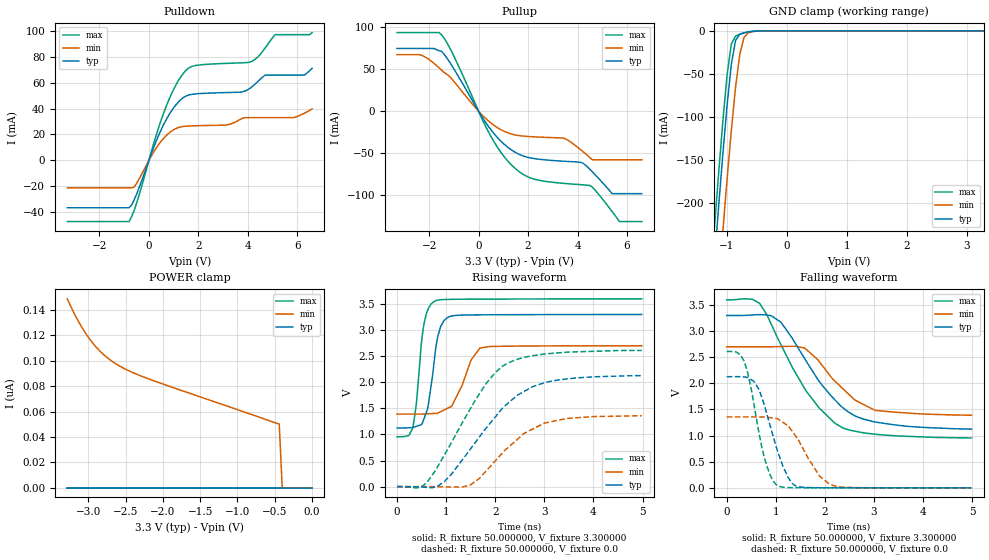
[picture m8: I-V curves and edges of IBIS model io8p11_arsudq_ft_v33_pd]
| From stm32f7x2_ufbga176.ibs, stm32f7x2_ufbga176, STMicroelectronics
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|   Model io8p11_arsudq_ft_v33_pd
[Model]  io8p11_arsudq_ft_v33_pd
Model_type I/O
Polarity   Non-Inverting
Enable   Active-Low
Vinl =   0.990000V
Vinh =   2.310000V
Vmeas =  1.650000V
Cref =   30.000000pF
Rref =   100.000000M
Vref =   0.0V
C_comp   2.292100pF   2.219400pF   2.369900pF
[Temperature Range]   25.000000   0.125000k   -40.000000
[Pullup Reference]   3.300000V   2.700000V   3.600000V
[Pulldown Reference]   0.0V   0.0V   0.0V
[POWER Clamp Reference]   3.300000V   2.700000V   3.600000V
[GND Clamp Reference]   0.0V   0.0V   0.0V
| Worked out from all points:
|   slope of the pulldown table from 0 to 0.495 V, typ, clamps not added: 20.9 ohm
|   slope of the pullup table from 0 to 0.495 V, typ, clamps not added: 22.6 ohm
|   GND clamp passes 1 mA (typ) near -0.62 V on its own axis
|   rising waveform, R_fixture 50.000000, V_fixture 3.300000: 20-80 % time 192ps typ, 344ps min, 163ps max; typ from 1.12 V to 3.3 V
|   rising waveform, R_fixture 50.000000, V_fixture 0.0: 20-80 % time 1.13ns typ, 939ps min, 1ns max; typ from 0 V to 2.13 V
|   falling waveform, R_fixture 50.000000, V_fixture 3.300000: 20-80 % time 999ps typ, 803ps min, 996ps max; typ from 3.3 V to 1.12 V
|   falling waveform, R_fixture 50.000000, V_fixture 0.0: 20-80 % time 415ps typ, 530ps min, 330ps max; typ from 2.13 V to 0 V
[Pulldown]
|Voltage   I(typ)   I(min)   I(max)
-3.3V     -36.46mA   -21.1mA    -47.09mA
-800mV    -36.46mA   -21.1mA    -47.09mA
-600mV    -30.5mA    -20.54mA   -38.69mA
700mV     31.4mA     19.11mA    41.71mA
1.2V      45.15mA    25.37mA    61.75mA
1.6V      50.35mA    26.5mA     71.06mA
3.1V      52.27mA    27.26mA    74.75mA
4.1V      55.69mA    32.97mA    75.8mA
4.7V      65.7mA     32.97mA    86.63mA
5.1V      65.7mA     32.97mA    96.89mA
6.3V      65.87mA    36.5mA     96.89mA
6.6V      70.93mA    39.71mA    98.5mA
[Pullup]
|Voltage   I(typ)   I(min)   I(max)
-3.3V     74.73mA    67.41mA    93.64mA
-2.3V     74.73mA    66.57mA    93.64mA
-1.5V     71.36mA    49.01mA    91.06mA
-1V       50.51mA    35.49mA    65.51mA
500mV     -22.07mA   -14mA      -30.03mA
1.6V      -50.64mA   -28.81mA   -70.96mA
3.5V      -59.53mA   -32.65mA   -85.92mA
4.2V      -61.43mA   -47.47mA   -87.46mA
4.5V      -69.06mA   -55.01mA   -88.38mA
5.4V      -98mA      -57.7mA    -119.3mA
5.7V      -98mA      -57.7mA    -131.2mA
6.6V      -98mA      -57.7mA    -131.2mA
[GND_clamp]
|Voltage   I(typ)   I(min)   I(max)
-3.3V     -2.314A    -2.394A    -2.287A
-1.2V     -265.5mA   -356.1mA   -227.2mA
-1.13V    -202.7mA   -292.9mA   -164.1mA
-1.06V    -142.2mA   -231.2mA   -104.1mA
-990mV    -85.98mA   -171.6mA   -50.73mA
-920mV    -38.81mA   -115.5mA   -15.29mA
-850mV    -11.09mA   -65.61mA   -6.016mA
-780mV    -3.793mA   -27.42mA   -3.89mA
-710mV    -2.098mA   -7.698mA   -2.396mA
-640mV    -1.159mA   -2.127mA   -1.234mA
-570mV    -535.1uA   -807.4uA   -490.2uA
3.28V     81.28uA    57.87uA    93.98uA
[POWER_clamp]
|Voltage   I(typ)   I(min)   I(max)
-3.28V    0A         148.5nA    0A
-3.2V     0A         138.6nA    0A
-3.12V    0A         129.7nA    0A
-3.04V    0A         122nA      0A
-2.96V    0A         115.3nA    0A
-2.8V     0A         105.1nA    0A
-2.6V     0A         96.44nA    0A
-2.4V     0A         90.52nA    0A
-2.16V    0A         84.97nA    0A
-440mV    0A         50.04nA    0A
-400mV    0A         0A         0A
0V        0A         0A         0A
[Ramp]
| variable   typ   min   max
dV/dt_r  1.26618/1.12392n   0.80934/0.93457n   1.56192/1.00073n
dV/dt_f  1.28340/0.99053n   0.77868/0.79554n   1.57246/0.99434n
R_load = 50.000000
[Rising Waveform]
R_fixture= 50.000000
V_fixture= 3.300000
V_fixture_min= 2.700000
V_fixture_max= 3.600000
|time   V(typ)   V(min)   V(max)
0s        1.123V     1.391V     953.8mV
320.3ps   1.132V     1.39V      1.122V
550.6ps   1.305V     1.393V     3.124V
630.6ps   1.526V     1.397V     3.393V
750.8ps   2.348V     1.402V     3.544V
830.8ps   2.88V      1.409V     3.574V
961ps     3.185V     1.469V     3.585V
1.121ns   3.27V      1.554V     3.589V
1.692ns   3.292V     2.656V     3.593V
4.985ns   3.299V     2.699V     3.598V
[Rising Waveform]
R_fixture= 50.000000
V_fixture= 0.0
V_fixture_min= 0.0
V_fixture_max= 0.0
|time   V(typ)   V(min)   V(max)
0s        211.7uV    83uV       632.1uV
550.6ps   -11.3mV    -125.6uV   33.63mV
961ps     92.14mV    -4.256mV   600.2mV
1.491ns   716.3mV    30.14mV    1.49V
1.812ns   1.118V     297mV      1.973V
2.232ns   1.576V     724.6mV    2.355V
2.593ns   1.826V     1.023V     2.477V
3.013ns   1.994V     1.22V      2.542V
3.473ns   2.066V     1.308V     2.577V
4.985ns   2.127V     1.358V     2.61V
[Falling Waveform]
R_fixture= 50.000000
V_fixture= 3.300000
V_fixture_min= 2.700000
V_fixture_max= 3.600000
|time   V(typ)   V(min)   V(max)
0s        3.299V     2.699V     3.598V
520.5ps   3.308V     2.699V     3.608V
670.7ps   3.314V     2.699V     3.53V
1.101ns   3.172V     2.704V     2.746V
1.592ns   2.467V     2.672V     1.893V
1.882ns   2.04V      2.418V     1.53V
2.362ns   1.536V     1.899V     1.148V
2.613ns   1.376V     1.679V     1.083V
3.023ns   1.26V      1.483V     1.027V
4.985ns   1.123V     1.391V     953.8mV
[Falling Waveform]
R_fixture= 50.000000
V_fixture= 0.0
V_fixture_min= 0.0
V_fixture_max= 0.0
|time   V(typ)   V(min)   V(max)
0s        2.127V     1.358V     2.61V
360.4ps   2.121V     1.357V     2.409V
560.6ps   2.027V     1.357V     1.566V
740.7ps   1.657V     1.356V     672.5mV
880.9ps   1.199V     1.342V     253.1mV
1.041ns   688.4mV    1.32V      40.77mV
1.381ns   48.73mV    1.02V      3.313mV
1.892ns   2.727mV    224.8mV    1.903mV
2.102ns   1.927mV    64.94mV    1.722mV
4.985ns   211.7uV    83uV       632.1uV
